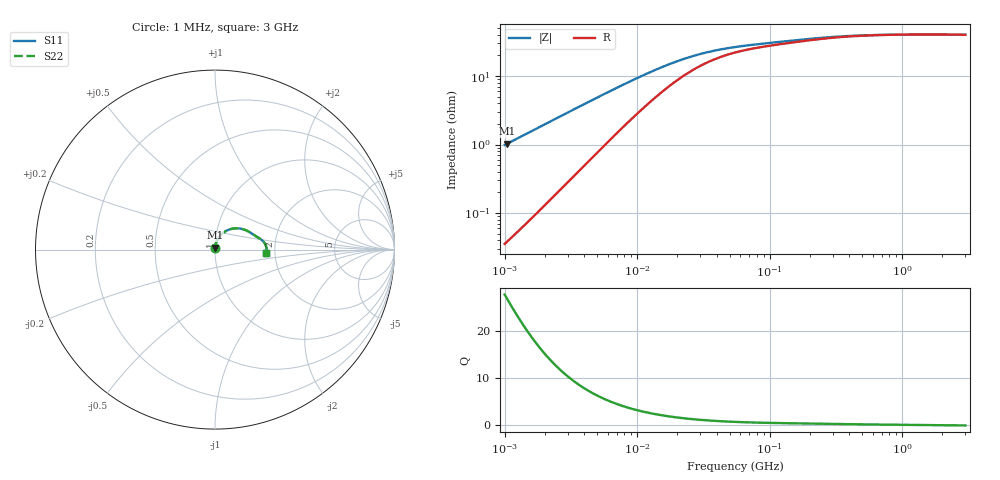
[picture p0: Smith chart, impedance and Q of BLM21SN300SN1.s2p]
! BLM21SN300SN1
# Hz S RI R 50
!Freq.(Hz) S11(Real) S11(Imag) S21(Real) S21(Imag) S12(Real) S12(Imag) S22(Real) S22(Imag)
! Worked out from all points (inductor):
!   401 points, 1 MHz to 3 GHz, reference 50 ohm
!   read as one part in series: L = 156 nH near 1.041 MHz
!   highest Q = 27 at 1.041 MHz (marker M1), where L = 156 nH
!   self-resonance near 1.487 GHz
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1000000  0.00045 0.00982  0.9996 -0.00982  0.9996 -0.00982  0.00045 0.00982
1040844  0.000484 0.0102  0.9995 -0.0102  0.9995 -0.0102  0.000484 0.0102
2097170  0.00183 0.0205  0.9982 -0.0205  0.9982 -0.0205  0.00183 0.0205
3823119  0.00586 0.0366  0.9941 -0.0366  0.9941 -0.0366  0.00586 0.0366
5938264  0.0136 0.055  0.9864 -0.055  0.9864 -0.055  0.0136 0.055
8345207  0.0253 0.0731  0.9747 -0.0731  0.9747 -0.0731  0.0253 0.0731
1.126754e7  0.0421 0.0905  0.9579 -0.0905  0.9579 -0.0905  0.0421 0.0905
1.461624e7  0.0628 0.1046  0.9372 -0.1046  0.9372 -0.1046  0.0628 0.1046
1.71545e7  0.0782 0.1115  0.9218 -0.1115  0.9218 -0.1115  0.0782 0.1115
2.013356e7  0.0952 0.1163  0.9048 -0.1163  0.9048 -0.1163  0.0952 0.1163
2.316168e7  0.1108 0.1185  0.8892 -0.1185  0.8892 -0.1185  0.1108 0.1185
2.718395e7  0.1287 0.1185  0.8713 -0.1185  0.8713 -0.1185  0.1287 0.1185
3.190472e7  0.1459 0.1162  0.8541 -0.1162  0.8541 -0.1162  0.1459 0.1162
3.74453e7  0.1618 0.1118  0.8382 -0.1118  0.8382 -0.1118  0.1618 0.1118
4.483659e7  0.1775 0.1054  0.8225 -0.1054  0.8225 -0.1054  0.1775 0.1054
5.477226e7  0.1923 0.0975  0.8077 -0.0975  0.8077 -0.0975  0.1923 0.0975
8.679508e7  0.2179 0.0808  0.7821 -0.0808  0.7821 -0.0808  0.2179 0.0808
2.094008e8  0.2561 0.057  0.7439 -0.057  0.7439 -0.057  0.2561 0.057
3.894533e8  0.2759 0.0372  0.7241 -0.0372  0.7241 -0.0372  0.2759 0.0372
8.005644e8  0.2859 0.0154  0.7141 -0.0154  0.7141 -0.0154  0.2859 0.0154
1.519029e9  0.2879 -0.00051  0.7121 0.00051  0.7121 0.00051  0.2879 -0.00051
3e9  0.2862 -0.018  0.7138 0.018  0.7138 0.018  0.2862 -0.018
